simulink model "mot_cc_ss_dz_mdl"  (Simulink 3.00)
settings: Solver=ode45  StartTime=0.0  StopTime=10.0  RelTol=1e-6  AbsTol=1e-6
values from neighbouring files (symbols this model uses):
  a1 = K*(T_camp+2*tau1)    [mot_cc_ss_int.m]
  a2 = K*(T_camp-2*tau1)    [mot_cc_ss_int.m]
  b = Ic0*Ke/Wmax    (= 8.2054202412e-06)    [mot_cc_ss_int.m]    (also in mot_cc_ss_k.m; Regolatore_Rs_discreto.m = -h*alpha; mot_cc_ss.m)
  b1 = T_camp+2*tau2    [mot_cc_ss_int.m]
  b2 = T_camp-2*tau2    [mot_cc_ss_int.m]
  C0 = 0*N*m    (= 0)    [mot_cc_ss_int.m]    (also in mot_cc_ss_k.m; mot_cc_ss.m)
  Ia0 = 0    [mot_cc_ss_int.m]    (also in mot_cc_ss_k.m; mot_cc_ss.m)
  Ia_max = Imax    (= 93.6)    [mot_cc_ss_int.m]    (also in mot_cc_ss_k.m)
  J = 9.2775e-006    (= 9.2775e-06)    [mot_cc_ss_int.m]    (also in mot_cc_ss_k.m; mot_cc_ss.m)
  Ke = Cmax/Imax    (= 0.00651965811966)    [mot_cc_ss_int.m]    (also in mot_cc_ss_k.m; mot_cc_ss.m)
  L = 60*10^-6    (= 6e-05)    [mot_cc_ss_int.m]    (also in mot_cc_ss_k.m; mot_cc_ss.m)
  R = Vn/Imax    (= 0.128205128205)    [mot_cc_ss_int.m]    (also in mot_cc_ss_k.m; mot_cc_ss.m)
  Tcsim = T_sim/1000    (= 8.42051458616e-06)    [mot_cc_ss_int.m]    (also in mot_cc_ss_k.m = 0.0001; mot_cc_ss.m = 0.001)
  Th0 = 0    [mot_cc_ss_int.m]    (also in mot_cc_ss_k.m; mot_cc_ss.m)
  Vi_max = Vn    (= 12)    [mot_cc_ss_int.m]    (also in mot_cc_ss_k.m)
  W_ref = R0    (= 100)    [mot_cc_ss_int.m]    (also in mot_cc_ss_k.m = 1047.1975512)
  Wm0 = 0    [mot_cc_ss_int.m]    (also in mot_cc_ss_k.m; mot_cc_ss.m)
undefined symbols (not defined in the file or in its folder): T_camp

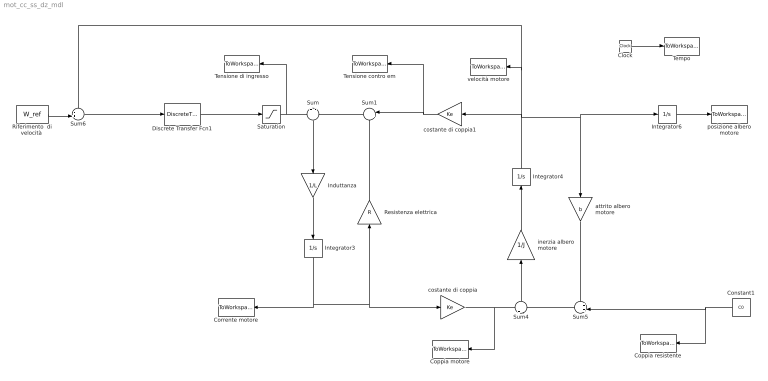
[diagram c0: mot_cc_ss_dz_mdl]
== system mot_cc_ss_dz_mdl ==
  Clock : Clock
  Constant1 : Constant  Orientation=left  Value=C0
  Coppia motore : ToWorkspace  VariableName=Cm  SampleTime=Tcsim  SaveFormat=Matrix
  Coppia resistente : ToWorkspace  VariableName=Cr  SampleTime=Tcsim  SaveFormat=Matrix
  Corrente motore : ToWorkspace  VariableName=Ia  SampleTime=Tcsim  SaveFormat=Matrix
  Discrete Transfer Fcn1 : DiscreteTransferFcn  Numerator=[a1 a2]  Denominator=[b1 b2]  SampleTime=T_camp
  Induttanza : Gain  Orientation=down  Gain=1/L  SaturateOnIntegerOverflow=on
  Integrator3 : Integrator  Orientation=down  ExternalReset=none  InitialConditionSource=internal  InitialCondition=Ia0  LimitOutput=on  UpperSaturationLimit=Ia_max  LowerSaturationLimit=-Ia_max  ShowSaturationPort=off  ShowStatePort=off  AbsoluteTolerance=auto
  Integrator4 : Integrator  Orientation=up  ExternalReset=none  InitialConditionSource=internal  InitialCondition=Wm0  LimitOutput=off  UpperSaturationLimit=inf  LowerSaturationLimit=-inf  ShowSaturationPort=off  ShowStatePort=off  AbsoluteTolerance=auto
  Integrator6 : Integrator  ExternalReset=none  InitialConditionSource=internal  InitialCondition=Th0  LimitOutput=off  UpperSaturationLimit=inf  LowerSaturationLimit=-inf  ShowSaturationPort=off  ShowStatePort=off  AbsoluteTolerance=auto
  Resistenza elettrica : Gain  Orientation=up  Gain=R  SaturateOnIntegerOverflow=on
  "Riferimento  di velocità " : Constant  Value=W_ref
  Saturation : Saturate  UpperLimit=Vi_max  LowerLimit=-Vi_max
  Sum : Sum  Orientation=down  Inputs=+|-  SaturateOnIntegerOverflow=on
  Sum1 : Sum  Orientation=left  Inputs=|++  SaturateOnIntegerOverflow=on
  Sum4 : Sum  Orientation=up  Inputs=+|-  SaturateOnIntegerOverflow=on
  Sum5 : Sum  Orientation=left  Inputs=++|  SaturateOnIntegerOverflow=on
  Sum6 : Sum  Inputs=-+|  SaturateOnIntegerOverflow=on
  Tempo : ToWorkspace  VariableName=t  SampleTime=Tcsim  SaveFormat=Matrix
  Tensione contro em : ToWorkspace  VariableName=E  SampleTime=Tcsim  SaveFormat=Matrix
  Tensione di ingresso : ToWorkspace  VariableName=Vi  SampleTime=Tcsim  SaveFormat=Matrix
  attrito albero motore : Gain  Orientation=down  Gain=b  SaturateOnIntegerOverflow=on
  costante di coppia : Gain  Gain=Ke  SaturateOnIntegerOverflow=on
  costante di coppia1 : Gain  Orientation=left  Gain=Ke  SaturateOnIntegerOverflow=on
  inerzia albero motore : Gain  Orientation=up  Gain=1/J  SaturateOnIntegerOverflow=on
  posizione albero motore : ToWorkspace  VariableName=Th  SampleTime=Tcsim  SaveFormat=Matrix
  velocità motore : ToWorkspace  VariableName=Wm  SampleTime=Tcsim  SaveFormat=Matrix
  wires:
  Sum/1 -> Induttanza/1
  Induttanza/1 -> Integrator3/1
  Sum1/1 -> Sum/2
  Integrator3/1 -> Corrente motore/1, costante di coppia/1, Resistenza elettrica/1
  Resistenza elettrica/1 -> Sum1/2
  Sum4/1 -> inerzia albero motore/1
  inerzia albero motore/1 -> Integrator4/1
  Sum5/1 -> Sum4/2
  attrito albero motore/1 -> Sum5/1
  Constant1/1 -> Coppia resistente/1, Sum5/2
  Integrator4/1 -> costante di coppia1/1, attrito albero motore/1, Integrator6/1, velocità motore/1, Sum6/1
  Integrator6/1 -> posizione albero motore/1
  costante di coppia/1 -> Sum4/1, Coppia motore/1
  costante di coppia1/1 -> Sum1/1, Tensione contro em/1
  Clock/1 -> Tempo/1
  Sum6/1 -> Discrete Transfer Fcn1/1
  Saturation/1 -> Sum/1, Tensione di ingresso/1
  "Riferimento  di velocità "/1 -> Sum6/2
  Discrete Transfer Fcn1/1 -> Saturation/1
